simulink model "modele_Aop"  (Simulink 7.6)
settings: Solver=ode45  StartTime=0.0  StopTime=10.0  RelTol=1e-3
libraries: powerlib x9

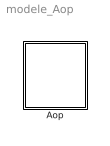
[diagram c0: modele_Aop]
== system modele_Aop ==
  Aop : Subsystem

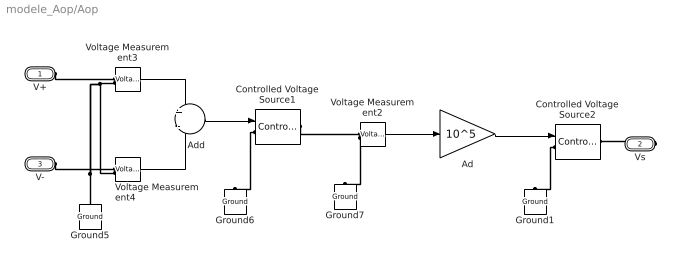
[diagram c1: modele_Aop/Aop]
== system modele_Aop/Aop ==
  Ad : Gain  Gain=10^5
  Add : Sum  Inputs=+-
  Controlled Voltage Source1 : powerlib/Electrical Sources/Controlled Voltage Source  DialogController=POWERSYS.PowerSysDialog  SystemSampleTime=-1  Initialize=on  Source_Type=AC  Amplitude=0  Phase=0  Frequency=0  Measurements=None
  Controlled Voltage Source2 : powerlib/Electrical Sources/Controlled Voltage Source  DialogController=POWERSYS.PowerSysDialog  SystemSampleTime=-1  Initialize=on  Source_Type=AC  Amplitude=0  Phase=0  Frequency=0  Measurements=None
  Ground{1,5..7} (4 alike) : powerlib/Elements/Ground  DialogController=POWERSYS.PowerSysDialog  PhysicalDomain=powersysdomain  SubClassName=unknown  LeftPortType=p1  RightPortType=p1  LConnTagsString=a
  Voltage Measurement2 : powerlib/Measurements/Voltage Measurement  DialogController=POWERSYS.PowerSysDialog  SystemSampleTime=-1  PhasorSimulation=off  OutputType=Complex  PSBequivalent=0
  Voltage Measurement3 : powerlib/Measurements/Voltage Measurement  DialogController=POWERSYS.PowerSysDialog  SystemSampleTime=-1  PhasorSimulation=off  OutputType=Complex  PSBequivalent=0
  Voltage Measurement4 : powerlib/Measurements/Voltage Measurement  DialogController=POWERSYS.PowerSysDialog  SystemSampleTime=-1  PhasorSimulation=off  OutputType=Complex  PSBequivalent=0
  V+ : PMIOPort  Port=1  Side=Left
  Vs : PMIOPort  Port=2  Side=Right
  V- : PMIOPort  Port=3  Side=Left
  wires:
  Add/1 -> Controlled Voltage Source1/1
  Voltage Measurement2/1 -> Ad/1
  Voltage Measurement4/1 -> Add/2
  Voltage Measurement3/1 -> Add/1
  Ad/1 -> Controlled Voltage Source2/1
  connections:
  Controlled Voltage Source1/LConn1 -- Ground6/LConn1
  Controlled Voltage Source1/RConn1 -- Voltage Measurement2/LConn1
  Controlled Voltage Source2/LConn1 -- Ground1/LConn1
  Voltage Measurement3/LConn2 -- Voltage Measurement4/LConn2 -- Ground5/LConn1
  Voltage Measurement2/LConn2 -- Ground7/LConn1
  V+/RConn1 -- Voltage Measurement3/LConn1
  Vs/RConn1 -- Controlled Voltage Source2/RConn1
  V-/RConn1 -- Voltage Measurement4/LConn1
